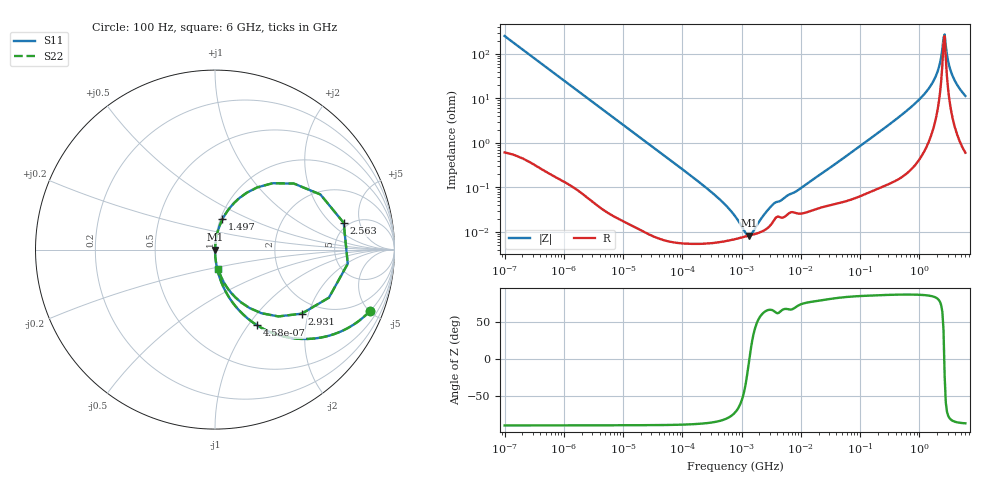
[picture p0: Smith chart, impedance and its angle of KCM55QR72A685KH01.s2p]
!Murata Part Number: KCM55QR72A685KH01
!These Parameters are Measured in Series Mode Connection
!Data Generated on Mar 13, 2026
!  o--ll--o
!Port1  Port2
!  o------o
!Operation Temp=25[degC], DC Bias Voltage=0[V]
!Freq. Start=100[Hz] Stop=6[GHz] 401[Steps]
# Hz S RI R 50
!Freq.(Hz) S11(Real) S11(Imag) S21(Real) S21(Imag) S12(Real) S12(Imag) S22(Real) S22(Imag)
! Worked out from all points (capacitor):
!   401 points, 100 Hz to 6 GHz, reference 50 ohm
!   read as one part in series: C = 6.29 uF near 109 Hz
!   lowest |Z| = 8.2 mohm at 1.326 MHz (marker M1)
!   series resonance near 1.353 MHz, so ESL is about 2.2 nH
!   S11 on the Smith chart (normalised r, x): 100 Hz: 1.01, -5.06; 458 Hz: 1.00, -1.11; 1.497 GHz: 1.02, +0.36; 2.563 GHz: 4.53, +2.92; 2.931 GHz: 1.62, -1.81; 6 GHz: 1.01, -0.23
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100  0.8641 -0.3415  0.1359 0.3415  0.1359 0.3415  0.8641 -0.3415
234  0.5391 -0.4966  0.4609 0.4966  0.4609 0.4966  0.5391 -0.4966
458  0.2356 -0.4222  0.7644 0.4222  0.7644 0.4222  0.2356 -0.4222
858  0.0819 -0.2717  0.9181 0.2717  0.9181 0.2717  0.0819 -0.2717
2008  0.0166 -0.1248  0.9834 0.1248  0.9834 0.1248  0.0166 -0.1248
40335  0.000111 -0.00638  0.9999 0.00638  0.9999 0.00638  0.000111 -0.00638
316350  5.65e-05 -0.000763  0.9999 0.000763  0.9999 0.000763  5.65e-05 -0.000763
774597  6.87e-05 -0.000216  0.9999 0.000216  0.9999 0.000216  6.87e-05 -0.000216
1108252  7.69e-05 -7.3e-05  0.9999 7.3e-05  0.9999 7.3e-05  7.69e-05 -7.3e-05
1325623  8.17e-05 -7.3e-06  0.9999 7.3e-06  0.9999 7.3e-06  8.17e-05 -7.3e-06
1585629  8.73e-05 5.76e-05  0.9999 -5.76e-05  0.9999 -5.76e-05  8.73e-05 5.76e-05
3394479  0.000169 0.000381  0.9998 -0.000381  0.9998 -0.000381  0.000169 0.000381
1.555665e7  0.000306 0.00144  0.9997 -0.00144  0.9997 -0.00144  0.000306 0.00144
3.124326e8  0.00187 0.0259  0.9981 -0.0259  0.9981 -0.0259  0.00187 0.0259
1.497423e9  0.0415 0.1686  0.9585 -0.1686  0.9585 -0.1686  0.0415 0.1686
1.95892e9  0.1364 0.2876  0.8636 -0.2876  0.8636 -0.2876  0.1364 0.2876
2.240541e9  0.3202 0.3696  0.6798 -0.3696  0.6798 -0.3696  0.3202 0.3696
2.562649e9  0.7171 0.1492  0.2829 -0.1492  0.2829 -0.1492  0.7171 0.1492
2.931063e9  0.4836 -0.3568  0.5164 0.3568  0.5164 0.3568  0.4836 -0.3568
3.205649e9  0.2583 -0.3543  0.7417 0.3543  0.7417 0.3543  0.2583 -0.3543
3.666503e9  0.1145 -0.2673  0.8855 0.2673  0.8855 0.2673  0.1145 -0.2673
6e9  0.0184 -0.1106  0.9816 0.1106  0.9816 0.1106  0.0184 -0.1106
